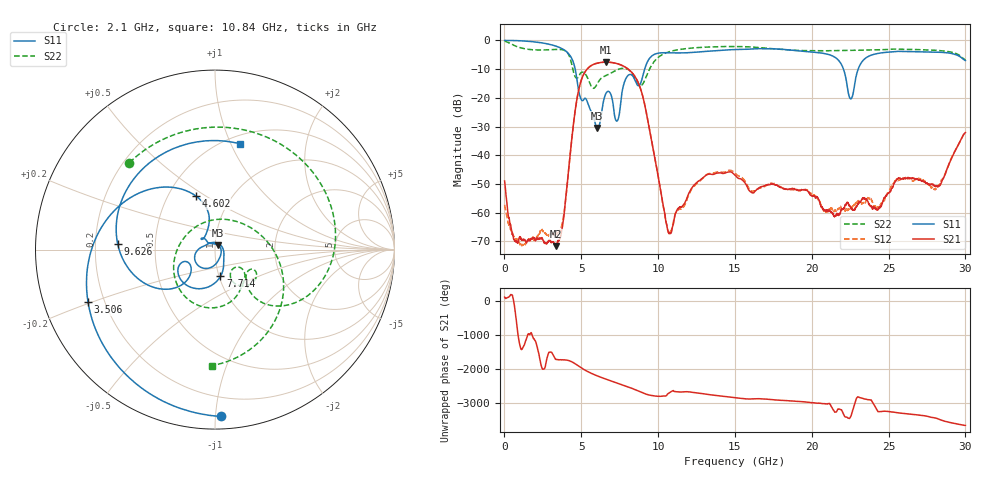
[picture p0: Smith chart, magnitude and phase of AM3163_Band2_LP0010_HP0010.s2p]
!Agilent Technologies,E8364B,MY43040894,A.07.50.67
!Agilent E8364B: A.07.50.67
!Date: Thursday, August 20, 2020 11:11:41
!Correction: S11(Full 2 Port(1,2))
!S21(Full 2 Port(1,2))
!S12(Full 2 Port(1,2))
!S22(Full 2 Port(1,2))
!S2P File: Measurements: S11, S21, S12, S22:
# Hz S  dB  R 50
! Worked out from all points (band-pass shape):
!   3201 points, 10 MHz to 30 GHz, reference 50 ohm
!   highest |S21| = -7.57 dB at 6.608 GHz (marker M1); lowest = -71.5 dB at 3.365 GHz (marker M2)
!   |S21| within 3 dB of the highest: 5.297 GHz to 8.175 GHz (2.878 GHz wide, 42.7 % of centre)
!   lowest |S11| = -30.5 dB at 6.045 GHz (marker M3), VSWR 1.06, Z = 51.6 + j2.57 ohm
!   |S11| at or under -10 dB: 4.604 GHz to 9.126 GHz (4.523 GHz wide, 65.9 % of centre); 22.06 GHz to 23.02 GHz (959.8 MHz wide, 4.26 % of centre)
!   |S22| runs from -16.7 to -0.3 dB; largest |S21 - S12| = 0.0049
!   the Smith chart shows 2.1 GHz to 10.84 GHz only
!   S11 on the Smith chart (normalised r, x): 2.1 GHz: 0.08, -1.03; 3.506 GHz: 0.14, -0.20; 4.602 GHz: 0.68, +0.45; 7.714 GHz: 1.02, -0.31; 9.626 GHz: 0.30, +0.03; 10.84 GHz: 0.58, +1.08
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1e7  -0.05 -2.8  -48.96 124.1  -57.23 -42.9  -0.28 -11.5
1.078394e9  -0.17 -44.4  -68.95 20.9  -71.57 -37.4  -2.64 -143.1
2.099928e9  -0.63 -88.0  -69.04 146.9  -68.54 -158.7  -3.35 134.5
3.365131e9  -2.04 -149.4  -71.55 82.8  -67.61 -22.5  -3.17 46.9
3.505709e9  -2.32 -157.4  -69.91 68.7  -67.33 -49.0  -3.16 36.2
4.602219e9  -9.96 109.7  -24.48 -50.4  -24.51 -50.8  -12.65 -42.3
5.014581e9  -20.74 128.2  -13.63 -175.8  -13.64 -176.0  -11.13 -34.8
6.045488e9  -30.52 56.7  -7.94 -50.7  -7.95 -50.9  -15.06 -35.3
6.6078e9  -18.45 -118.8  -7.57 -146.9  -7.57 -147.0  -12.24 -50.2
7.320062e9  -28.12 59.6  -8.08 100.0  -8.12 99.8  -10.31 -74.4
7.713681e9  -16.37 -78.4  -8.88 37.6  -8.93 37.7  -9.73 -96.5
9.625544e9  -5.31 176.7  -36.40 84.8  -36.36 84.1  -8.28 -16.2
1.000979e10  -4.47 142.1  -47.56 64.8  -47.32 63.2  -5.93 -46.4
1.084389e10  -4.35 76.7  -66.99 -158.5  -66.48 170.9  -3.79 -91.4
1.227778e10  -4.20 -18.0  -50.78 178.2  -51.00 -179.0  -2.65 -144.5
1.5005e10  -3.18 -143.8  -46.93 20.0  -46.18 18.6  -2.15 127.2
1.769473e10  -2.99 94.0  -50.36 -45.5  -50.18 -48.5  -3.02 28.2
2.000958e10  -4.08 -29.8  -54.07 -123.9  -53.57 -122.1  -3.63 -51.8
2.253999e10  -20.36 -105.2  -58.05 -178.8  -58.35 -96.5  -3.52 -122.5
2.500479e10  -4.12 -151.4  -53.17 -27.5  -52.82 -21.9  -3.19 177.5
2.811625e10  -4.11 111.9  -50.73 134.2  -51.29 128.1  -3.48 95.0
3e10  -7.04 41.6  -32.10 -78.9  -32.10 -79.1  -6.82 37.4
